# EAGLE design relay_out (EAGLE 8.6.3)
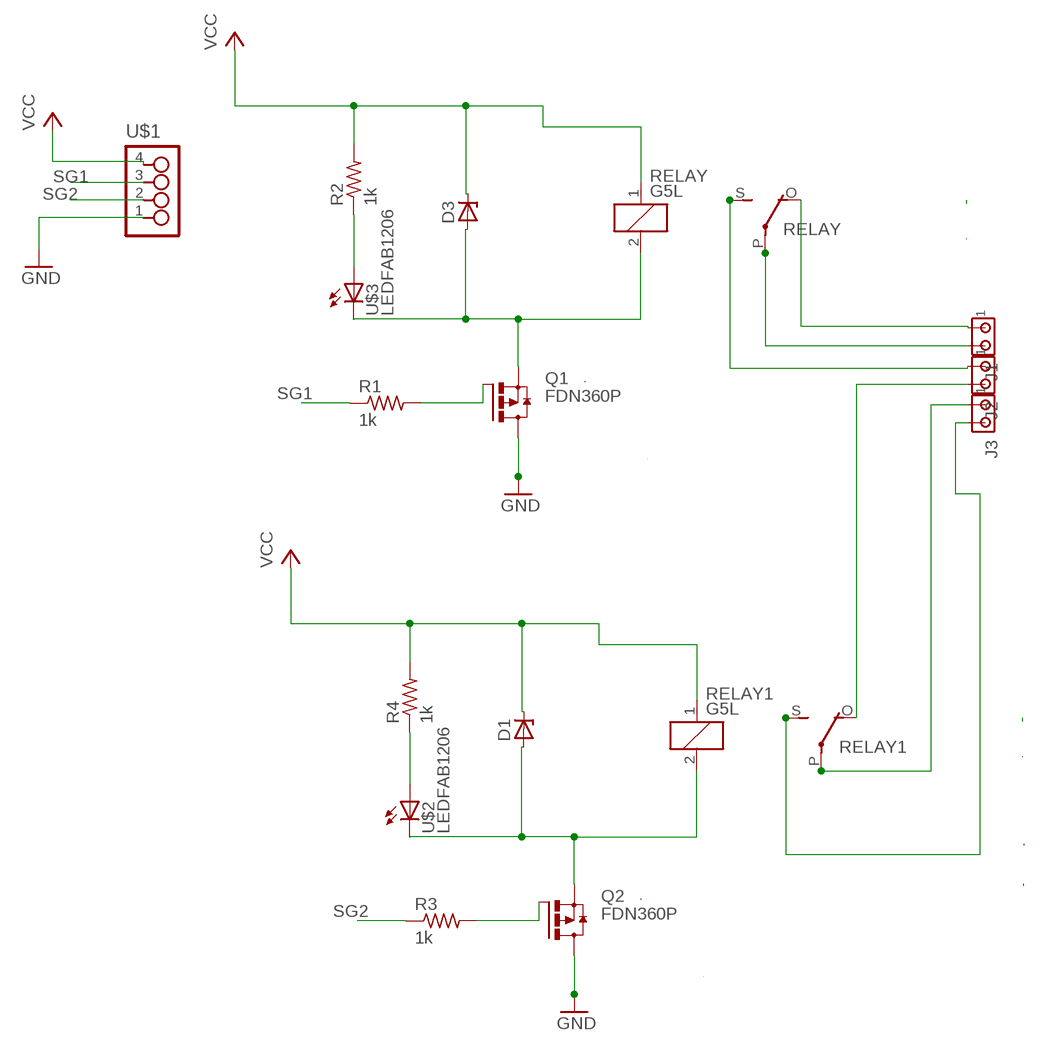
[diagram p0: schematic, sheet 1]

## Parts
D1  ZENER_DIODESOD123  [SOD123]
D3  ZENER_DIODESOD123  [SOD123]
J1  MTA02-156  [1X2MTA]
J2  MTA02-156  [1X2MTA]
J3  MTA02-156  [1X2MTA]
Q1  FDN360P  [SUPER-SOT3]
Q2  FDN360P  [SUPER-SOT3]
R1  1k  RES-US1206FAB  [R1206FAB]
R2  1k  RES-US1206FAB  [R1206FAB]
R3  1k  RES-US1206FAB  [R1206FAB]
R4  1k  RES-US1206FAB  [R1206FAB]
RELAY  G5L  [G5LE]
RELAY1  G5L  [G5LE]
U$1  4_PIN_HEADERHEADER  [SMT_PINS_4]
U$2  LEDFAB1206  [LED1206FAB]
U$3  LEDFAB1206  [LED1206FAB]

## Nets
GND: Q1.3(D) Q2.3(D) U$1.1
N$2: Q1.1(G) R1.2
N$3: D1.ANODE Q2.2(S) RELAY1.2 U$2.2(C)
N$4: D3.ANODE Q1.2(S) RELAY.2 U$3.2(C)
N$5: R2.1 U$3.1(A)
N$6: J1.1 RELAY.O(2:O)
N$8: R4.1 U$2.1(A)
N$16: J2.1 RELAY.S(2:S)
N$17: J1.2 RELAY.P(2:P)
N$19: Q2.1(G) R3.2
N$20: J3.2 RELAY1.S(2:S)
N$21: J3.1 RELAY1.P(2:P)
N$22: J2.2 RELAY1.O(2:O)
SG1: R1.1 U$1.3
SG2: R3.1 U$1.2
VCC: D1.CATHODE D3.CATHODE R2.2 R4.2 RELAY1.1 RELAY.1 U$1.4

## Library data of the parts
D1 D3 = fab:ZENER_DIODE: zener diode
J1-J3 = con-amp:MTA02-156: AMP connector
Q1 Q2 = transistor-power:FDN360P: Single P-Channel, PowerTrench (R) MOSFET Source: http://www.fairchildsemi.com/ds/FD/FDN360P.pdf
R1-R4 = fab:RES-US: Resistor (US Symbol)
RELAY RELAY1 = relay:G5L: RELAY 1 x switch, 10 A/120 V AC, 8 A/30 V ADC, Omron
U$1 = FabLab:4_PIN_HEADER: 4 SMT pin pads
U$2 U$3 = fab:LED: LED

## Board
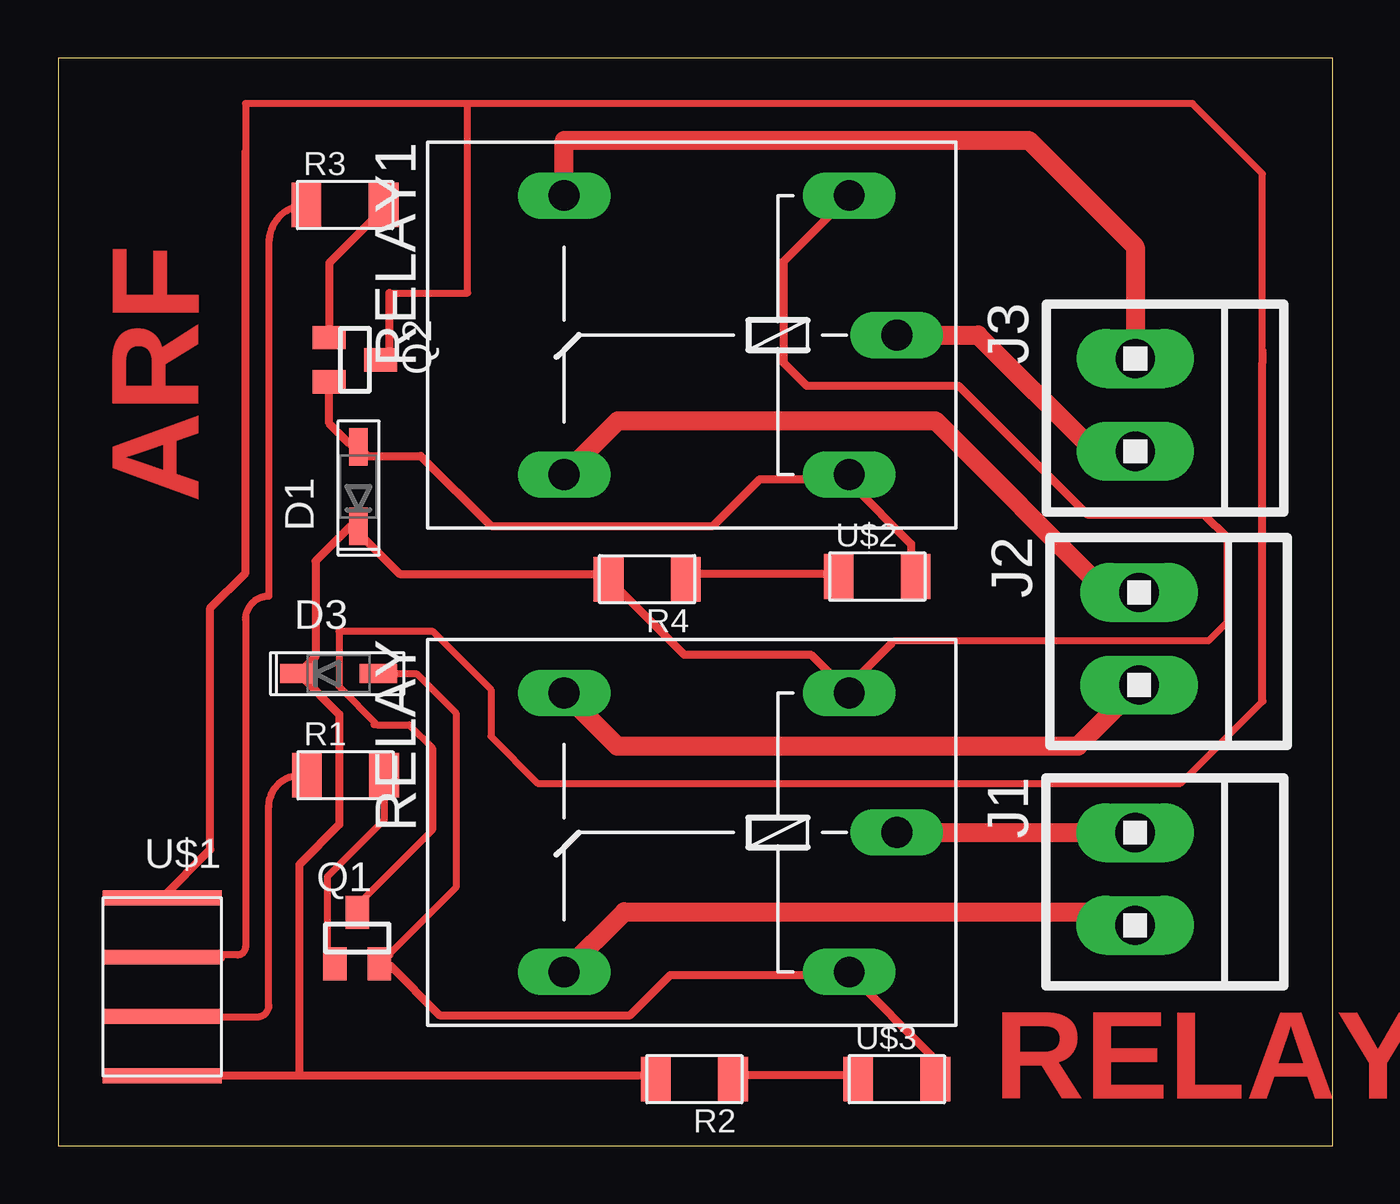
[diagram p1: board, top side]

Size 54.5 x 46.5 mm. Coordinates in mm from the lower left corner, seen from the top.
Outline: 0,0 54.5,0 54.5,46.5 0,46.5 0,0
Copper layers (1*16): Top 0.035mm / dielectric 1.5mm / Bottom 0.035mm
Design rules "default *": minimum track width 0.35mm, minimum drill 0.35mm, track to track 20mil, track to pad 10mil, pad to pad 6mil, via to via 6mil, smd to smd 6mil, copper to edge 70mil, drill to drill 6mil, minimum pad ring 10mil, minimum via ring 8mil, stop-mask expansion 4mil, vias tented up to drill 0mil, thermal gap 10mil

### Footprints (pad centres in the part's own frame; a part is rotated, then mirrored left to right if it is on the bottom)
SOD123 = smd 1.6 x 0.8: ANODE 1.7,0; CATHODE -1.7,0
1X2MTA = drill 1.676 long: 1 1.981,0; 2 -1.981,0
SUPER-SOT3 = smd 1 x 1.4: 1 -0.95,-1.1; 2 0.95,-1.1; 3 0,1.1
R1206FAB = smd 1.27 x 1.905: 1 -1.651,0; 2 1.651,0
G5LE = drill 1.321 long: 1 -7.493,-5.969; 2 -7.493,5.969; O 4.699,5.969; P -9.525,0; S 4.699,-5.969
SMT_PINS_4 = smd 5.08 x 0.635: 1 0,0; 2 0,2.54; 3 0,5.08; 4 0,7.62
LED1206FAB = smd 1.27 x 1.905: 1 -1.651,0; 2 1.651,0

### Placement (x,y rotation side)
D1  12.83,28.19 90 top
D3  11.98,20.19 0 top
J1  46.05,11.4 270 top
J2  46.22,21.68 270 top
J3  46.06,31.68 270 top
Q1  12.78,8.87 0 top
Q2  12.68,33.61 270 top
R1  12.28,15.84 0 top
R2  27.2,2.84 180 top
R3  12.26,40.23 0 top
R4  25.18,24.23 180 top
RELAY  26.33,13.39 180 top
RELAY1  26.33,34.67 180 top
U$1  4.44,10.6 180 top
U$2  35.02,24.34 0 top
U$3  35.86,2.84 0 top

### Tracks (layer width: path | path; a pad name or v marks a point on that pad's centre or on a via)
GND
  Top 0.305: 13.64,18 13.5,18 | Q1.3 12.78,10.28 16,13.5 16,17 15,18 13.64,18 | 13.64,18 12,19.64 12,22 16,22 18.5,19.5 18.5,17.5 20.5,15.5 48,15.5 51.5,19 | 51.5,33.5 51.5,41.57 48.5,44.57 17.5,44.57 | 8,42 8,44.57 17.5,44.57 | 14.16,36.47 17.5,36.47 17.5,44.57
  Top 0.35: 14.16,36.47 14.16,33.89 Q2.3 | 12.87,10.3 Q1.3 | 4.72,10.72 U$1.1 6.5,12.66 6.5,23 8,24.5 8,42 8,42.5 | 51.5,34 51.5,33.5 51.5,19
N$2
  Top 0.305: R1.2 13.93,13.93 11.5,11.5 11.5,8.23 11.58,8.15
  Top 0.35: 11.58,8.15 Q1.1 | 13.73,15.44 R1.2
N$3
  Top 0.35: Q2.2 11.58,32.6 11.58,30.89 12.44,30.03 D1.ANODE | U$2.2 36.47,24.45 36.47,25.74 33.89,28.31 33.86,28.48 | 33.86,28.48 RELAY1.2 33.46,28.31 | 12.87,29.6 D1.ANODE | D1.ANODE 13.22,29.5 15.5,29.5 18.5,26.5 28,26.5 30,28.5 33.84,28.5 33.86,28.48
N$4
  Top 0.305: D3.ANODE 15.31,20.19 17,18.5 17,11.04 Q1.2
  Top 0.35: U$3.2 37.32,3 37.32,3.86 33.89,7.29 RELAY.2 33.46,7.29 26.17,7.29 24.45,5.58 16.3,5.58 14.16,7.72 Q1.2 14.16,8.15 | 13.73,20.16 D3.ANODE
N$5
  Top 0.35: R2.1 29.17,3 33.89,3 U$3.1
N$6
  Top 0.813: RELAY.O 24.21,10 45.47,10 J1.1
N$8
  Top 0.35: R4.1 27.03,24.45 33.03,24.45 U$2.1
N$16
  Top 0.813: RELAY.S 23.9,17.09 43.61,17.09 J2.1
N$17
  Top 0.813: RELAY.P J1.2
N$19
  Top 0.35: Q2.1 11.58,34.75 11.58,37.75 13.73,39.9 R3.2
N$20
  Top 0.813: RELAY1.S 21.63,43 41.5,43 46.06,38.44 J3.2
N$21
  Top 0.35: 45.9,30.03 J3.1
  Top 0.813: RELAY1.P 39.33,34.67 44.3,29.7 J3.1
N$22
  Top 0.813: RELAY1.O 23.93,31 37.5,31 44.84,23.66 J2.2
SG1
  Top 0.305: U$1.3 arc90 4.46,5.5 8.5,5.5 arc90 9,6 9,14.5 arc-90 10.34,15.84 R1.1
  Top 0.35: 5.58,5.58 4.72,5.58 U$1.3 | 10.3,15.44 R1.1
SG2
  Top 0.254: 7,8 6.85,8.15 5.5,8.15
  Top 0.305: R3.1 arc90 9,38.62 9,23.5 arc90 8,22.5 8,8.5 arc-90 7.65,8.15 5,8.15
  Top 0.35: 5.58,8.15 5.5,8.15 5,8.15 4.72,8.15 U$1.2 | 10.3,39.9 R3.1
VCC
  Top 0.305: 35.61,21.45 35.76,21.6 49.2,21.6 50,22.4 50,22.8
  Top 0.35: 10.3,3 4.72,3 U$1.4 | 10.3,3 25.31,3 R2.2 | R4.2 23.17,24.45 14.59,24.45 12.87,26.17 D1.CATHODE 12.49,26.49 11,25 11,20.91 D3.CATHODE 10.3,20.16 12.01,18.45 12.01,13.73 10.3,12.01 10.3,3 | 23.59,24.02 R4.2 | 35.61,21.45 33.89,19.73 RELAY.1 32.18,21 26.76,21 R4.2 | 50,22.5 50,22.8 50,26 49,27 44,27 38.5,32.5 32,32.5 31,33.5 31,37.82 RELAY1.1

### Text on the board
Top: ARF | RELAY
